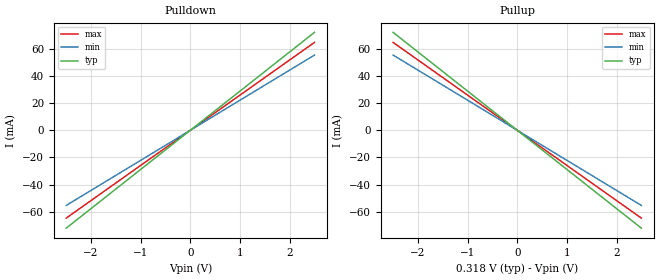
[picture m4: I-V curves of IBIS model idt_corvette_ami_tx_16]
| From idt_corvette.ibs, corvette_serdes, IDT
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|   model   idt_corvette_ami_tx_16
[Model] idt_corvette_ami_tx_16
Model_type Output
C_comp 400f 400f 400f
Cref = 0
[Model Spec]
Vmeas 0. 0. 0.
Vref 0. 0. 0.
[Temperature Range]  25 100 0
[Voltage Range] .318 .323 .276
[Algorithmic Model]
Executable Windows_VisualStudio5_32 idt_corvette_tx.dll   idt_corvette_tx.ami
Executable Windows_ver_64   idt_corvette_tx_64.dll   idt_corvette_tx.ami
Executable Linux_gcc4.1.2_32   idt_corvette_tx.linux.so   idt_corvette_tx.ami
Executable Linux_gcc3.2.3_64   idt_corvette_tx_64.linux.so idt_corvette_tx.ami
[End Algorithmic Model]
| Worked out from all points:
|   slope of the pulldown table from 0 to 0.048 V, typ, clamps not added: 34.8 ohm
|   slope of the pullup table from 0 to 0.048 V, typ, clamps not added: 34.8 ohm
[Pulldown]
-2.5V     -71.94mA   -55.25mA   -64.56mA
0V        0A         0A         0A
2.5V      71.94mA    55.25mA    64.56mA
[Pullup]
-2.5V     71.94mA    55.25mA    64.56mA
0V        0A         0A         0A
2.5V      -71.94mA   -55.25mA   -64.56mA
[Ramp]
dV/dt_r .113/19.46p .102/25.34p .0932/21.684p
dV/dt_f .113/19.46p .102/25.34p .0932/21.684p
